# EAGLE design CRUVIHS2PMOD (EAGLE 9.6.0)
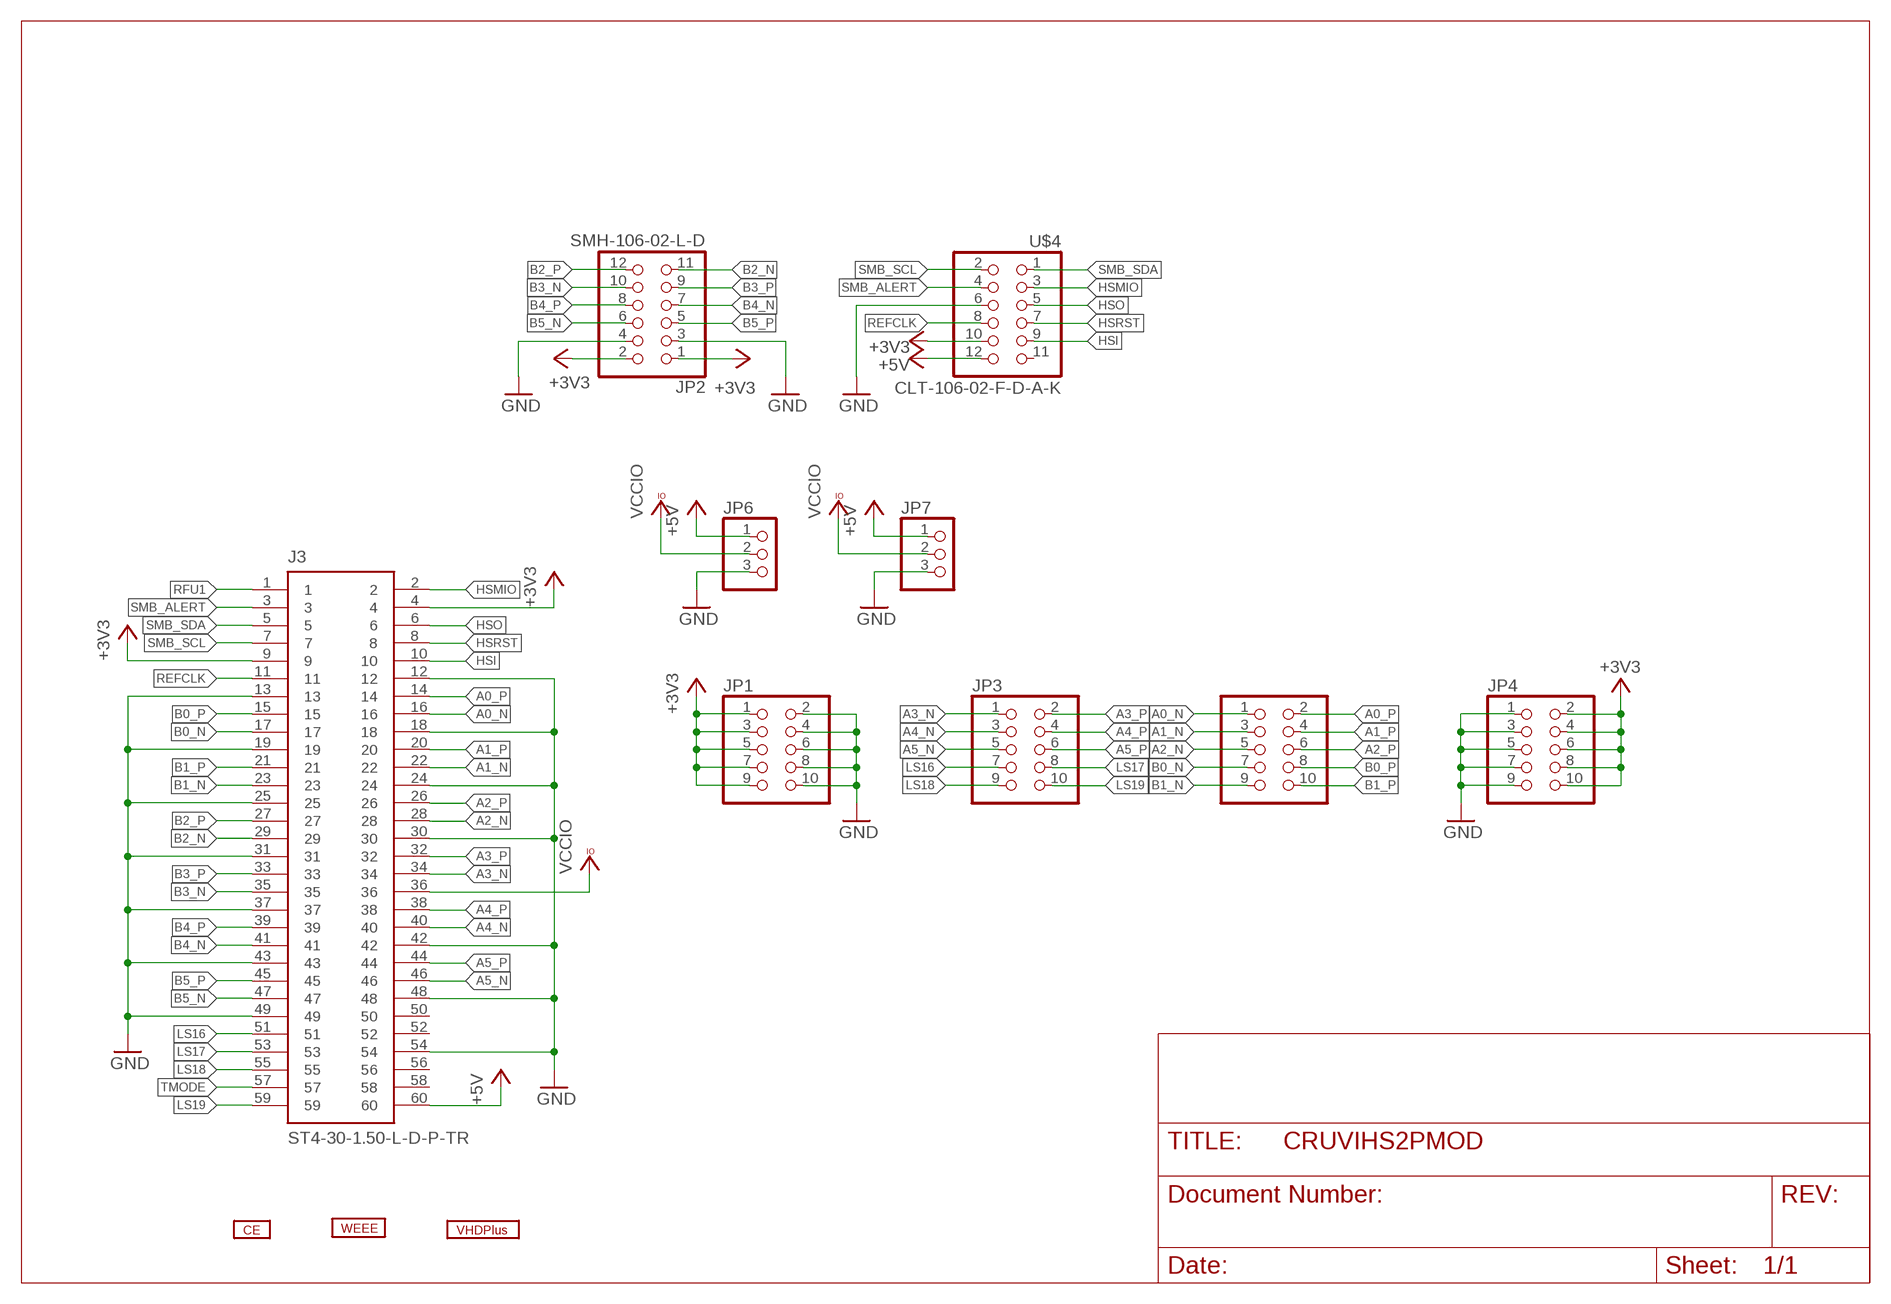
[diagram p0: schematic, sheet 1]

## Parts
J3  ST4-30-1.50-L-D-P-TR  [SAMTEC_ST4-30-1.50-L-D-P-TR]
JP1  PINHD-2X5  [2X05]
JP2  SMH-106-02-L-D  PINHD-2X6_2.54-SMD-90°  [2X06SMD/90]
JP3  PINHD-2X5  [2X05]
JP4  PINHD-2X5  [2X05]
JP5  PINHD-2X5  [2X05]
JP6  PINHD-1X3_2.54  [1X03]
JP7  PINHD-1X3_2.54  [1X03]
U$1  CE  [CE]
U$2  WEEE  [WEEE]
U$3  VHDPLUS_S_TEXT  [VHDPLUS_XS_TEXT]
U$4  CLT-106-02-F-D-A-K  [CLT-106-02-F-D-A-K]

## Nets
+3V3: J3.4 J3.9 JP1.1 JP1.3 JP1.5 JP1.7 JP1.9 JP2.1 JP2.2 JP4.2 JP4.4 JP4.6 JP4.8 JP4.10 U$4.10
+5V: J3.60 JP6.1 JP7.1 U$4.12
A0_N: J3.16 JP5.1
A0_P: J3.14 JP5.2
A1_N: J3.22 JP5.3
A1_P: J3.20 JP5.4
A2_N: J3.28 JP5.5
A2_P: J3.26 JP5.6
A3_N: J3.34 JP3.1
A3_P: J3.32 JP3.2
A4_N: J3.40 JP3.3
A4_P: J3.38 JP3.4
A5_N: J3.46 JP3.5
A5_P: J3.44 JP3.6
B0_N: J3.17 JP5.7
B0_P: J3.15 JP5.8
B1_N: J3.23 JP5.9
B1_P: J3.21 JP5.10
B2_N: J3.29 JP2.11
B2_P: J3.27 JP2.12
B3_N: J3.35 JP2.10
B3_P: J3.33 JP2.9
B4_N: J3.41 JP2.7
B4_P: J3.39 JP2.8
B5_N: J3.47 JP2.6
B5_P: J3.45 JP2.5
GND: J3.12 J3.13 J3.18 J3.19 J3.24 J3.25 J3.30 J3.31 J3.37 J3.42 J3.43 J3.48 J3.49 J3.54 JP1.2 JP1.4 JP1.6 JP1.8 JP1.10 JP2.3 JP2.4 JP4.1 JP4.3 JP4.5 JP4.7 JP4.9 JP6.3 JP7.3 U$4.6
HSI: J3.10 U$4.9
HSMIO: J3.2 U$4.3
HSO: J3.6 U$4.5
HSRST: J3.8 U$4.7
LS16: J3.51 JP3.7
LS17: J3.53 JP3.8
LS18: J3.55 JP3.9
LS19: J3.59 JP3.10
REFCLK: J3.11 U$4.8
RFU1: J3.1
SMB_ALERT: J3.3 U$4.4
SMB_SCL: J3.7 U$4.2
SMB_SDA: J3.5 U$4.1
TMODE: J3.57
VCCIO: J3.36 JP6.2 JP7.2
Unconnected: J3.50 J3.52 J3.56 J3.58 U$4.11

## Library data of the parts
J3 = ST4-30-1.50-L-D-P-TR:ST4-30-1.50-L-D-P-TR: ST4 Series 0.40 mm Micro Blade & Beam Ultra Fine Pitch Terminal Strip; AVAILABILITY: Unavailable; DESCRIPTION: 60 Position Connector Header, Center Strip Contacts Surface Mount Gold; MF: Samtec; MP: ST4-30-1.50-L-D-P-TR; PACKAGE: None; PRICE: None
JP1 JP3-JP5 = pinhead:PINHD-2X5: PIN HEADER
JP2 = pinhead2:PINHD-2X6: PIN HEADER
JP6 JP7 = pinhead2:PINHD-1X3: PIN HEADER
U$1 = VHDP_LOGO:CE
U$2 = VHDP_LOGO:WEEE
U$3 = VHDPlus_Logo:VHDPLUS_S_TEXT
U$4 = CLT-106-02-F-D-A-K:CLT-106-02-F-D-A-K

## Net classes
1 diff pairs: width 0.152 mm

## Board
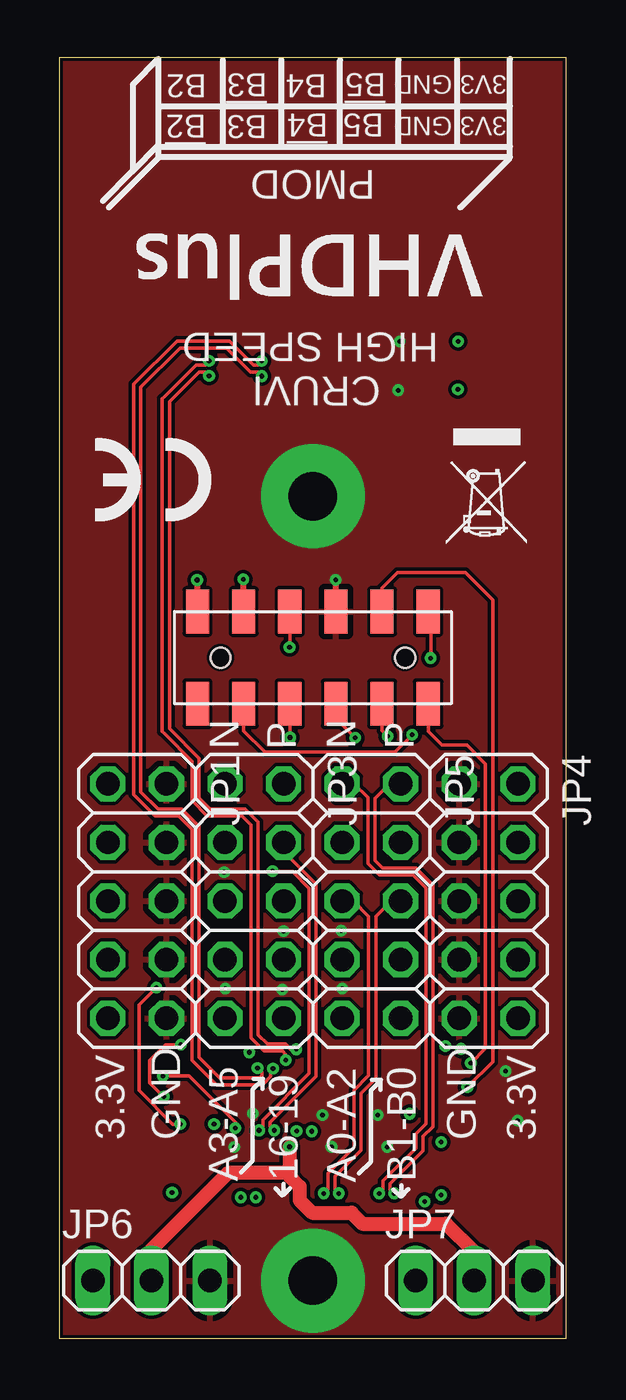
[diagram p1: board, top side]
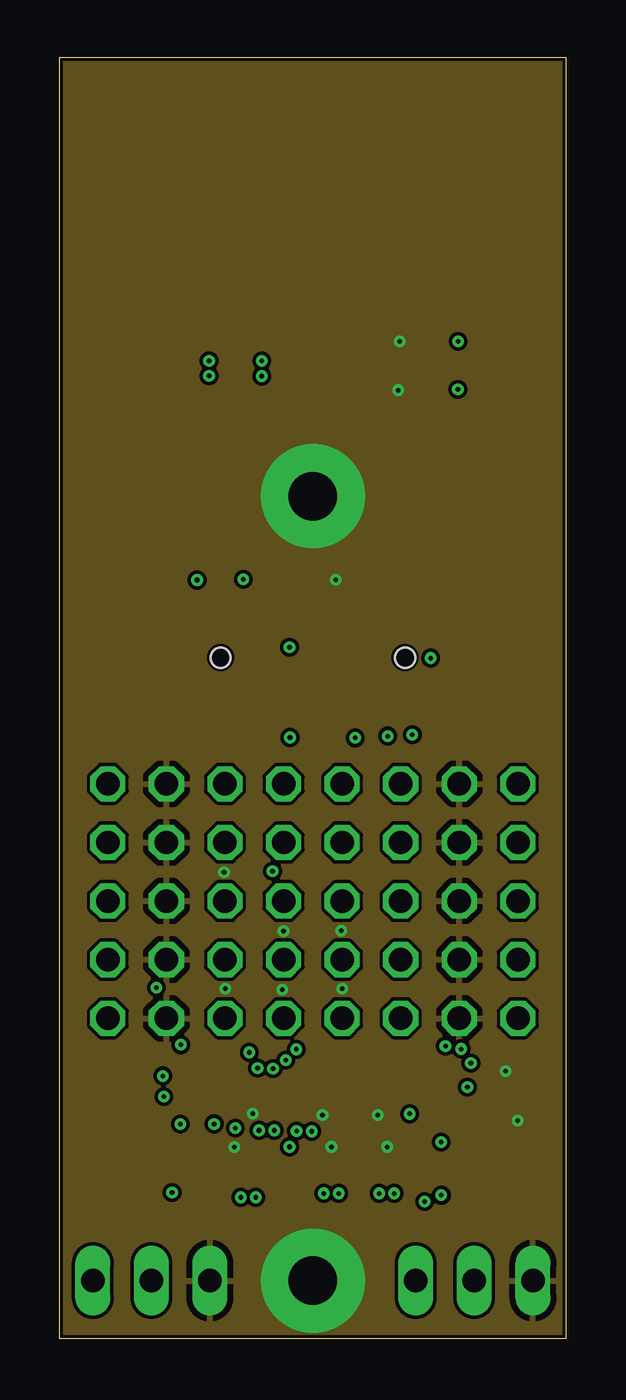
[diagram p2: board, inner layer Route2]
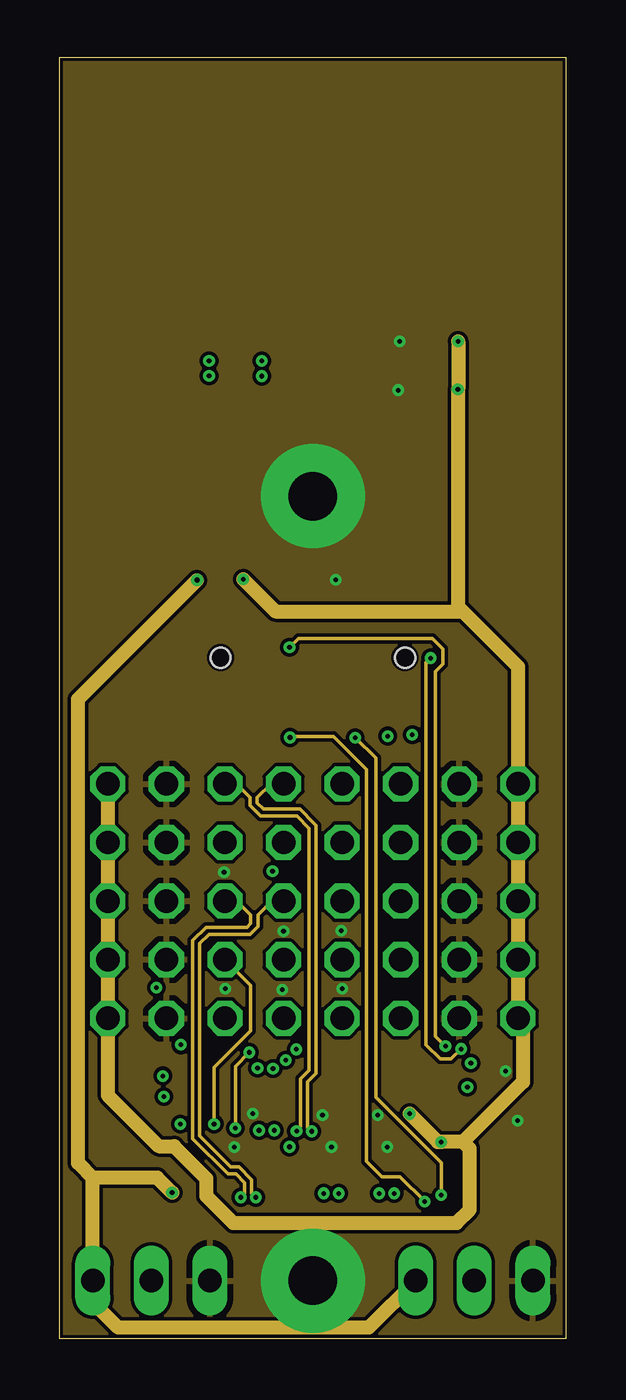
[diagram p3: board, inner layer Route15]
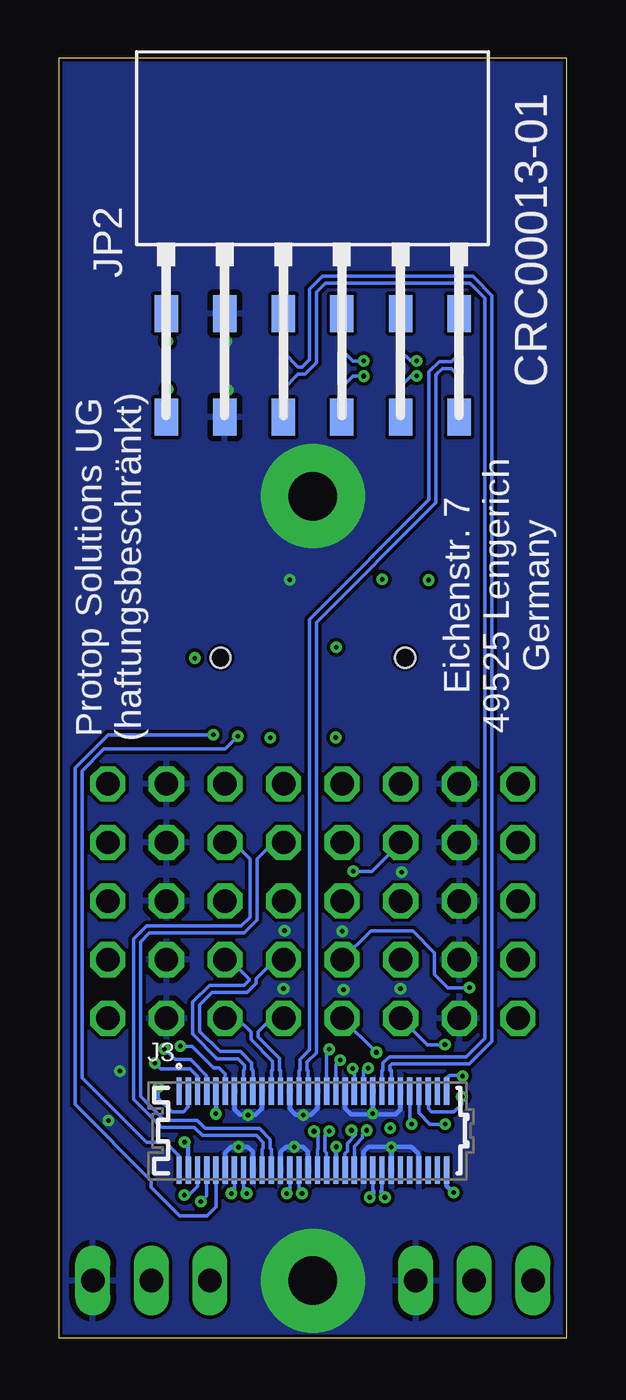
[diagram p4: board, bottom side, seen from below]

Size 22 x 55.5 mm. Coordinates in mm from the lower left corner, seen from the top.
Outline: 0,0 22,0 22,55.5 0,55.5 0,0
Copper layers (1+2*15+16): Top 0.035mm / dielectric 1.5mm / Route2 0.035mm / dielectric 0.15mm / Route15 0.035mm / dielectric 0.2mm / Bottom 0.035mm
Design rules "default *": minimum track width 6mil, minimum drill 0.2mm, track to track 6mil, track to pad 6mil, pad to pad 6mil, via to via 6mil, smd to smd 0mil, copper to edge 6mil, drill to drill 6mil, minimum pad ring 6mil, minimum via ring 6mil, stop-mask expansion 4mil, vias tented up to drill 15mil, thermal gap 10mil

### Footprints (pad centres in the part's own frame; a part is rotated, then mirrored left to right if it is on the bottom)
SAMTEC_ST4-30-1.50-L-D-P-TR = smd 0.23 x 1.2: 1 -5.8,1.71; 2 -5.8,-1.71; 3 -5.4,1.71; 4 -5.4,-1.71; 5 -5,1.71; 6 -5,-1.71; 7 -4.6,1.71; 8 -4.6,-1.71; 9 -4.2,1.71; 10 -4.2,-1.71; 11 -3.8,1.71; 12 -3.8,-1.71; 13 -3.4,1.71; 14 -3.4,-1.71; 15 -3,1.71; 16 -3,-1.71; 17 -2.6,1.71; 18 -2.6,-1.71; 19 -2.2,1.71; 20 -2.2,-1.71; 21 -1.8,1.71; 22 -1.8,-1.71; 23 -1.4,1.71; 24 -1.4,-1.71; 25 -1,1.71; 26 -1,-1.71; 27 -0.6,1.71; 28 -0.6,-1.71; 29 -0.2,1.71; 30 -0.2,-1.71; 31 0.2,1.71; 32 0.2,-1.71; 33 0.6,1.71; 34 0.6,-1.71; 35 1,1.71; 36 1,-1.71; 37 1.4,1.71; 38 1.4,-1.71; 39 1.8,1.71; 40 1.8,-1.71; 41 2.2,1.71; 42 2.2,-1.71; 43 2.6,1.71; 44 2.6,-1.71; 45 3,1.71; 46 3,-1.71; 47 3.4,1.71; 48 3.4,-1.71; 49 3.8,1.71; 50 3.8,-1.71; 51 4.2,1.71; 52 4.2,-1.71; 53 4.6,1.71; 54 4.6,-1.71; 55 5,1.71; 56 5,-1.71; 57 5.4,1.71; 58 5.4,-1.71; 59 5.8,1.71; 60 5.8,-1.71
2X05 = drill 1.016 octagon: 1 -5.08,-1.27; 2 -5.08,1.27; 3 -2.54,-1.27; 4 -2.54,1.27; 5 0,-1.27; 6 0,1.27; 7 2.54,-1.27; 8 2.54,1.27; 9 5.08,-1.27; 10 5.08,1.27
2X06SMD/90 = smd 1.02 x 1.6: 1 -1.27,-9.844; 2 -1.27,-5.344; 3 1.27,-9.844; 4 1.27,-5.344; 5 3.81,-9.844; 6 3.81,-5.344; 7 6.35,-9.844; 8 6.35,-5.344; 9 8.89,-9.844; 10 8.89,-5.344; 11 11.43,-9.844; 12 11.43,-5.344
1X03 = drill 1.016 long: 1 -2.54,0; 2 0,0; 3 2.54,0
CLT-106-02-F-D-A-K = smd 1.02 x 1.9: 1 -5,2 | smd 1 x 1.9: 2 -5,-2; 3 -3,2; 4 -3,-2; 5 -1,2; 6 -1,-2; 7 1,2; 8 1,-2; 9 3,2; 10 3,-2; 11 5,2; 12 5,-2 | hole 0.87: -4,0; 4,0

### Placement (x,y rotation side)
J3  11,9 0 bottom
JP1  3.38,18.95 270 top
JP2  16.09,49.76 0 bottom
JP3  8.46,18.95 270 top
JP4  18.62,18.95 270 top
JP5  13.54,18.95 270 top
JP6  4,2.5 0 top
JP7  18,2.5 0 top
U$1  4.17,37.19 180 top
U$2  18.57,36.34 180 top
U$3  18.5,48 180 top
U$4  11,29.5 180 top

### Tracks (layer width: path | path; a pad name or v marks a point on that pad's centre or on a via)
+3V3  (via drill 0.2)
  Top 0.254: U$4.10 v8,32.88 v7.99,32.89
  Route15 0.61: v17.3,43.2 v17.3,41.13 v17.29,41.12 17.29,31.71 17.5,31.5 | v7.99,32.89 9.38,31.5 17.5,31.5 | 17.5,31.5 19.89,29.11 JP4.2 JP4.4 JP4.6 JP4.8 JP4.10 20.11,13.65 20.11,11.11 17.51,8.51 | 17.51,8.51 v16.56,8.51 16.42,8.51 v15.2,9.73 | JP1.1 JP1.3 JP1.5 JP1.7 JP1.9 2.11,10.53 4.32,8.32 4.99,8.32 6.38,6.93 6.38,6.17 7.55,5 17.23,5 17.8,5.57 17.8,8.22 17.51,8.51
  Bottom 0.203: v16.56,8.51 16.4,8.35 J3.4 | J3.9 v15.2,9.73
  Bottom 0.254: JP2.1 17.36,41.05 v17.29,41.12 | JP2.2 17.3,44.36 v17.3,43.2
+5V  (via drill 0.2)
  Top 0.254: U$4.12 6,32.84 v5.98,32.86
  Route15 0.61: v4.9,6.31 4.25,6.96 1.46,6.96 | v5.98,32.86 0.82,27.7 0.82,7.6 1.46,6.96 | 1.46,6.96 JP6.1 1.46,1.56 2.56,0.46 13.42,0.46 JP7.1
  Bottom 0.203: J3.60 5.2,6.61 v4.9,6.31
A0_N  (via drill 0.2)
  Top 0.152: v13.87,6.28 14.05,6.46 14.05,6.82 15.47,8.24 15.47,8.87 15.9,9.3 15.9,19.52 15.34,20.08 13.89,20.08 13.38,20.58 13.38,23.43 12.79,24.03 JP5.1
  Bottom 0.152: J3.16 14,6.38 13.89,6.28 v13.87,6.28
A0_P  (via drill 0.2)
  Top 0.152: v14.53,6.28 14.35,6.46 14.35,6.69 15.78,8.12 15.78,8.74 16.2,9.18 16.2,19.65 15.47,20.39 14.02,20.39 13.69,20.71 13.69,23.39 14.33,24.03 JP5.2
  Bottom 0.152: J3.14 14.4,6.38 14.51,6.28 v14.53,6.28
A1_N
  Bottom 0.152: J3.22 12.8,8.2 12.85,8.24 12.85,8.63 13.32,9.1 15.66,9.1 16.02,9.46 17.43,9.46 18.47,10.49 18.47,17.18 18.09,17.56 13.98,17.56 13.41,18.12 13.41,20.78 12.71,21.49 JP5.3
A1_P
  Bottom 0.152: J3.20 13.2,8.2 13.15,8.24 13.15,8.5 13.44,8.79 15.79,8.79 16.15,9.15 17.56,9.15 18.77,10.36 18.77,17.31 18.22,17.86 14.11,17.86 13.72,18.25 13.72,20.77 14.44,21.49 JP5.4
A2_N  (via drill 0.2)
  Top 0.152: v11.47,6.28 11.65,6.46 11.65,7.15 12.78,8.28 12.78,10.75 13.42,11.39 13.42,18.29 12.76,18.95 JP5.5
  Bottom 0.152: J3.28 11.6,6.38 11.49,6.28 v11.47,6.28
A2_P  (via drill 0.2)
  Top 0.152: v12.13,6.28 11.95,6.46 11.95,7.02 13.09,8.15 13.09,10.62 13.73,11.28 13.73,18.28 14.4,18.95 JP5.6
  Bottom 0.152: J3.26 12,6.38 12.11,6.28 v12.13,6.28
A3_N  (via drill 0.2)
  Route15 0.152: v10.29,8.98 10.47,9.16 10.47,11.24 10.83,11.61 10.83,22.11 10.31,22.63 8.74,22.63 8.29,23.08 8.29,23.43 7.68,24.03 JP3.1
  Bottom 0.152: J3.34 10.4,8.03 10.47,8.1 10.47,8.8 v10.29,8.98
A3_P  (via drill 0.2)
  Route15 0.152: v10.95,8.97 10.78,9.15 10.78,11.12 11.05,11.39 | 11.05,11.39 | 11.05,11.39 11.14,11.48 11.14,22.23 11.05,22.32 | 11.05,22.32 | JP3.2 9.19,24.03 8.59,23.43 8.59,23.21 8.87,22.93 10.44,22.93 11.05,22.32
  Bottom 0.152: J3.32 10.8,8.2 10.78,8.22 10.78,8.79 v10.95,8.97
A4_N  (via drill 0.2)
  Top 0.152: v8.67,9.01 8.85,9.19 8.85,9.48 10.84,11.47 10.84,19.5 10.11,20.23 v9.26,20.23 v9.25,20.24
  Bottom 0.152: J3.40 9.2,8.33 8.85,8.69 8.85,8.83 v8.67,9.01 | v9.25,20.24 8.44,20.24 JP3.3
A4_P  (via drill 0.2)
  Top 0.152: v9.33,9.01 9.15,9.19 9.15,9.35 11.14,11.35 11.14,19.69 9.73,21.1 JP3.4
  Bottom 0.152: J3.38 9.6,8.01 9.51,8.1 9.51,8.45 9.15,8.81 9.15,8.83 v9.33,9.01
A5_N  (via drill 0.2)
  Route15 0.152: v7.87,6.11 8.05,6.29 8.05,6.74 7.67,7.12 7.31,7.12 5.79,8.64 5.79,17.24 6.37,17.82 8.15,17.82 8.31,17.97 8.31,18.34 7.7,18.95 JP3.5
  Bottom 0.152: J3.46 8,6.38 8.05,6.38 8.05,6.29 v7.87,6.11
A5_P  (via drill 0.2)
  Route15 0.152: v8.53,6.11 8.35,6.29 8.35,6.87 7.79,7.42 7.44,7.42 6.1,8.77 6.1,17.11 6.5,17.51 8.28,17.51 8.62,17.84 8.62,18.34 9.22,18.95 JP3.6
  Bottom 0.152: J3.44 8.4,6.38 8.35,6.38 8.35,6.29 v8.53,6.11
B0_N
  Bottom 0.152: J3.17 13.6,11.62 13.65,11.66 13.65,11.95 14.13,12.43 15.03,12.43 15.91,13.31 15.91,14.45 15.36,15 13.85,15 13.46,15.38 13.46,15.57 12.62,16.41 JP5.7
B0_P
  Bottom 0.152: J3.15 14,11.62 13.95,11.66 13.95,11.82 14.25,12.12 15.15,12.12 16.21,13.18 16.21,14.58 15.49,15.3 13.97,15.3 13.77,15.51 13.77,15.57 14.61,16.41 JP5.8
B1_N
  Bottom 0.152: J3.23 12.4,11.62 12.45,11.62 12.45,12.14 13.38,13.07 13.38,13.28 12.79,13.87 JP5.9
B1_P
  Bottom 0.152: J3.21 12.8,11.62 12.75,11.62 12.75,12.01 13.69,12.95 13.69,13.28 14.28,13.87 JP5.10
B2_N
  Bottom 0.152: J3.29 11.2,11.62 11.25,11.62 11.25,11.97 10.85,12.38 10.85,31.02 5.66,36.22 5.66,41.77 5.39,42.03 5,42.03 4.66,41.69 JP2.11
B2_P
  Bottom 0.152: J3.27 11.6,11.62 11.55,11.62 11.55,12.1 11.15,12.5 11.15,31.15 5.96,36.34 5.96,41.89 5.52,42.34 5,42.34 4.66,42.67 JP2.12
B3_N  (via drill 0.2)
  Top 0.152: v9.82,12.06 9.82,12.31 9.68,12.45 8.89,12.45 8.32,13.02 8.32,22.25 7.92,22.64 6.42,22.64 5.77,23.3 5.77,25.01 4.56,26.21 | 4.56,26.21 | 4.56,26.21 4.47,26.3 4.47,40.73 4.56,40.82 | 4.56,40.82 | v6.5,42.36 6.5,42.33 6.36,42.19 5.93,42.19 4.56,40.82
  Bottom 0.152: v9.82,12.06 10,11.88 J3.35 | JP2.10 7.2,42.79 6.77,42.36 v6.5,42.36
B3_P  (via drill 0.2)
  Top 0.152: v10.29,12.53 10.04,12.53 9.8,12.76 9.03,12.76 8.62,13.15 8.62,22.38 8.05,22.95 6.55,22.95 6.08,23.43 6.08,25.14 4.78,26.43 4.78,40.6 6.06,41.88 6.36,41.88 6.5,41.74 v6.5,41.7
  Bottom 0.152: v10.29,12.53 10.4,12.41 J3.33 | JP2.9 7.2,41.25 6.75,41.7 v6.5,41.7
B4_N  (via drill 0.2)
  Top 0.152: v8.6,11.71 8.8,11.52 8.8,11.41 8.68,11.29 6.95,11.29 6.06,12.18 6.06,22.18 5.31,22.93 4.29,22.93 3.54,23.68 3.54,41.22 5.24,42.92 7.26,42.92 8.3,41.88 8.61,41.88 v8.79,41.7
  Bottom 0.152: v8.6,11.71 8.7,11.71 8.8,11.62 8.8,11.47 J3.41 | JP2.7 9.74,41.22 9.26,41.7 v8.79,41.7
B4_P  (via drill 0.2)
  Top 0.152: v9.28,11.68 9.18,11.58 9.18,11.35 8.9,11.07 | 8.9,11.07 | 8.9,11.07 8.81,10.98 6.82,10.98 6.73,11.07 | 6.73,11.07 | 6.73,11.07 5.75,12.05 5.75,22.05 5.18,22.63 4.16,22.63 3.23,23.56 3.23,41.35 5.11,43.23 7.39,43.23 8.43,42.18 8.61,42.18 v8.79,42.36
  Bottom 0.152: J3.39 9.2,11.62 v9.27,11.68 v9.28,11.68 | JP2.8 9.74,42.84 9.26,42.36 v8.79,42.36
B5_N
  Bottom 0.152: J3.47 7.6,11.62 7.65,11.62 7.65,11.8 7.56,11.89 4.22,11.89 3.23,12.87 3.23,45.2 3.97,45.94 | 3.97,45.94 | 3.97,45.94 4.06,46.02 10.59,46.02 10.68,45.94 | 10.68,45.94 | JP2.6 12.28,42.73 11.64,42.09 11.46,42.09 11.14,42.41 11.14,45.47 10.68,45.94
B5_P
  Bottom 0.152: J3.45 8,11.62 7.95,11.62 7.95,11.93 7.69,12.2 4.34,12.2 3.54,13 3.54,45.07 4.19,45.72 10.46,45.72 10.84,45.34 10.84,42.28 11.33,41.78 11.64,41.78 12.28,41.15 JP2.5
GND  (via drill 0.2, 2.1 pad 4.5)
  Top 0.254: U$4.6 v12,32.88
  Bottom 0.203: J3.13 14.4,9.92 14.16,9.68 v13.81,9.68 13.48,9.68 13.2,9.96 J3.19 | J3.25 12,9.94 11.75,9.69 v11.43,9.69 v11.42,9.68 v11.41,9.69 11.07,9.69 10.8,9.96 J3.31 | J3.37 9.6,9.96 9.36,9.71 8.38,9.71 | J3.43 v8.4,9.73 8.38,9.71 | J3.49 7.2,9.92 7.41,9.71 8.29,9.71 8.38,9.71 | J3.12 14.8,8.04 14.54,8.29 v14.22,8.29 14.21,8.3 13.83,8.3 13.6,8.07 J3.18 | J3.24 12.4,8.07 12.17,8.3 11.82,8.3 v11.81,8.29 11.8,8.3 11.42,8.3 11.2,8.08 J3.30 | J3.42 8.8,8.07 8.58,8.29 8.24,8.29 v7.6,8.29 | v7.6,8.29 J3.48 | J3.54 6.43,7.32 6.43,8 6.73,8.29 v7.6,8.29
  Bottom 0.254: JP2.4 14.82,43.27 v14.76,43.21 | JP2.3 14.82,40.97 v14.7,41.09
  other vias: 11,2.5 11,36.5 12.23,17.66 12.27,15.15 19.36,11.58 19.87,9.43 9.67,15.11 9.73,17.65 7.2,15.15 7.15,20.2
  pour Route2: 0,-0.1 22.05,-0.1 22.05,55.45 0,55.45
  pour Top: 0,0 0,55.5 22,55.5 22,0
  pour Route15: 0,0 22,0 22,55.5 0,55.5
  pour Bottom: 0,0 22,0 22,55.5 0,55.5
HSI  (via drill 0.2)
  Top 0.152: U$4.9 8,26.33 8.92,25.41 14.57,25.41 v15.31,26.15
  Bottom 0.152: J3.10 15.2,5.69 15.59,5.3 16.77,5.3 18.01,6.54 18.01,6.83 21.31,10.13 21.31,24.72 19.88,26.15 v15.31,26.15
HSMIO  (via drill 0.2)
  Top 0.152: U$4.3 14,26.35 v14.25,26.1
  Bottom 0.152: v14.25,26.1 14.81,25.54 20.06,25.54 21,24.59 21,11.3 18.2,8.49 17.39,8.49 16.8,7.9 J3.2
HSO  (via drill 0.2)
  Top 0.152: v12.84,26.02 12,26.86 U$4.5
  Route15 0.152: v12.84,26.02 v12.85,26.02 13.73,25.14 13.73,10.45 16.57,7.61 v16.57,6.2
  Bottom 0.152: J3.6 16,6.58 16.38,6.2 v16.57,6.2
HSRST  (via drill 0.2)
  Top 0.152: v10.01,26.04 U$4.7
  Route15 0.152: v10.01,26.04 10.06,26.09 11.89,26.09 13.33,24.65 13.33,9.88 13.33,7.67 14,7 14.78,7 v15.85,5.93
  Bottom 0.152: J3.8 15.6,6.18 v15.85,5.93
LS16  (via drill 0.2)
  Route15 0.152: JP3.7 8.3,15.3 8.3,13.32 6.72,11.74 v6.72,9.29
  Bottom 0.152: J3.51 6.8,9.37 v6.72,9.29
LS17  (via drill 0.2)
  Top 0.152: v4.21,15.19 3.47,14.45 3.47,10.74 4.93,9.28 v5.26,9.28
  Bottom 0.152: JP3.8 8.48,17.66 6.67,17.66 5.72,16.71 5.72,15.77 5.14,15.19 v4.21,15.19 | J3.53 6.4,9.76 5.92,9.28 v5.26,9.28
LS18  (via drill 0.2)
  Top 0.152: v5.27,12.72 4.61,12.72 3.93,12.04 3.93,11.08 v4.54,10.47
  Bottom 0.152: J3.55 6,9.96 5.85,9.81 4.88,9.81 4.55,10.14 v4.55,10.46 v4.54,10.47 | JP3.9 6.04,12.72 v5.27,12.72
LS19  (via drill 0.2)
  Top 0.152: v4.5,11.37 5.63,11.37 7.64,9.36 v7.64,9.11
  Route15 0.152: v8.24,12.39 7.64,11.79 v7.64,9.11
  Bottom 0.152: J3.59 5.2,11.29 5.09,11.4 4.53,11.4 v4.5,11.37 | JP3.10 v8.25,12.39 v8.24,12.39
REFCLK  (via drill 0.2)
  Top 0.152: U$4.8 v10,29.96 v9.99,29.95
  Route15 0.152: v16.75,12.66 16.32,13.09 16.32,28.9 16.64,29.22 16.64,29.88 16.19,30.33 10.37,30.33 v9.99,29.95
  Bottom 0.152: J3.11 14.8,11.47 15.06,11.73 15.31,11.73 16.24,12.66 v16.75,12.66
SMB_ALERT  (via drill 0.2)
  Top 0.152: v17.7,10.89 18.8,11.99 18.8,32 17.62,33.18 14.67,33.18 14,32.51 U$4.4
  Bottom 0.152: J3.3 16.4,10.02 16.61,9.81 17.11,9.81 17.7,10.4 v17.7,10.89
SMB_SCL  (via drill 0.2)
  Top 0.152: v16.11,29.48 16.11,31.39 U$4.2
  Route15 0.152: v17.43,12.54 16.99,12.1 16.53,12.1 15.91,12.72 15.91,29.28 v16.11,29.48
  Bottom 0.152: J3.7 15.6,11.38 16.31,12.09 16.98,12.09 v17.43,12.54
SMB_SDA  (via drill 0.2)
  Top 0.152: v17.85,11.92 18.49,12.56 18.49,24.89 17.67,25.71 16.59,25.71 16,26.3 U$4.1
  Bottom 0.152: J3.5 16,11.35 16.32,11.67 17.6,11.67 v17.85,11.92
VCCIO  (via drill 0.2)
  Top 0.203: 9.99,7.01 v9.99,8.3
  Top 0.61: JP6.2 4,3.85 7.32,7.17 9.99,7.17 v9.99,8.3 | JP7.2 18,3.74 16.77,4.97 13.15,4.97 12.68,5.44 10.97,5.44 10.43,5.98 10.43,6.57 9.99,7.01
  Bottom 0.203: v9.99,8.3 v10,8.29 J3.36

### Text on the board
tPlace: B2 | !B3 | B4 | !B5 | GND | 3V3 | !B2 | B3 | !B4 | B5 | GND | 3V3 | PMOD | CRUVI / HIGH SPEED | N | P | N | P | 3.3V | GND | GND | 3.3V | A3-A5 | 16-19 | A0-A2 | B1-B0
bPlace: CRC00013-01 | Protop Solutions UG / (haftungsbeschränkt) | Eichenstr. 7 / 49525 Lengerich / Germany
